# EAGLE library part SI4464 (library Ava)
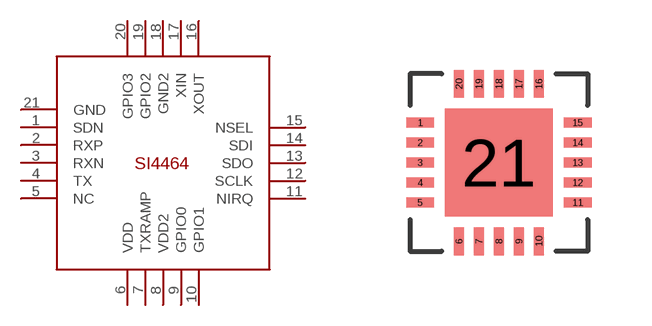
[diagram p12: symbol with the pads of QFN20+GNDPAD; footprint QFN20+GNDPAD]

Designator prefix -

## SI4464  [QFN20+GNDPAD]
1  SDN
2  RXP
3  RXN
4  TX
5  NC
6  VDD
7  TXRAMP
8  VDD2
9  GPIO0
10  GPIO1
11  NIRQ
12  SCLK
13  SDO
14  SDI
15  NSEL
16  XOUT
17  XIN
18  GND2
19  GPIO2
20  GPIO3
21  GND

## Footprint QFN20+GNDPAD (pad centres in mm)
smd 0.7 x 0.25: 1 -1.97,1; 2 -1.97,0.5; 3 -1.97,0; 4 -1.97,-0.5; 5 -1.97,-1; 11 1.97,-1; 12 1.97,-0.5; 13 1.97,0; 14 1.97,0.5; 15 1.97,1
smd 0.25 x 0.7: 6 -1,-1.97; 7 -0.5,-1.97; 8 0,-1.97; 9 0.5,-1.97; 10 1,-1.97; 16 1,1.97; 17 0.5,1.97; 18 0,1.97; 19 -0.5,1.97; 20 -1,1.97
smd 2.7 x 2.7: 21 0,0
